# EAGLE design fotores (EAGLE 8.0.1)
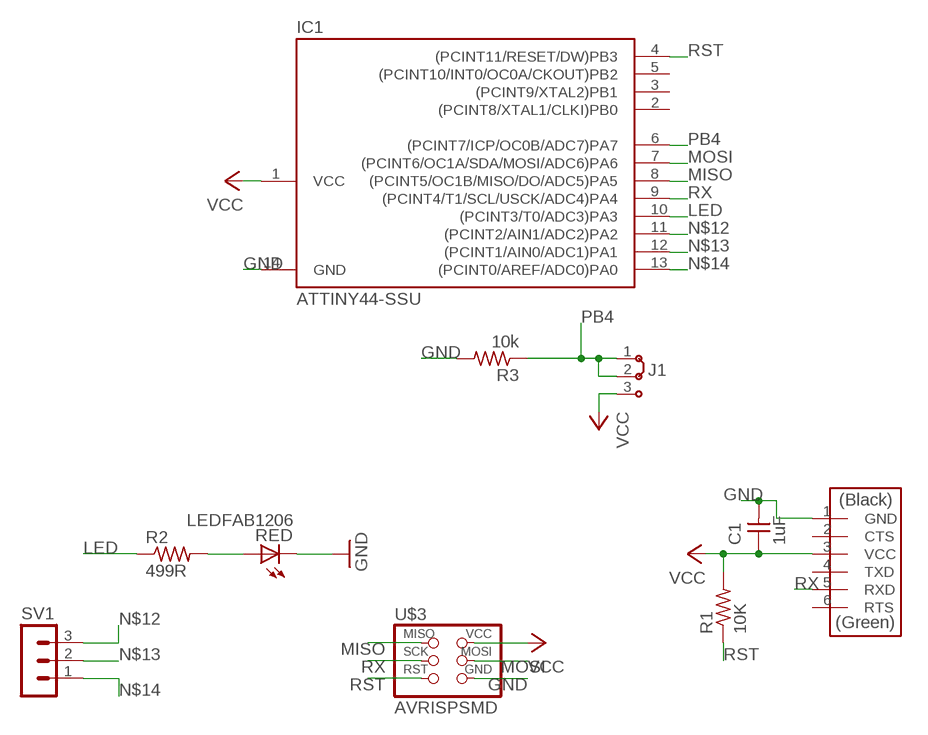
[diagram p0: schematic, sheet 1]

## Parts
C1  1uF  CAP-UNPOLARIZEDFAB  [C1206FAB]
IC1  ATTINY44-SSU  [SOIC14]
J1  J2X2MM  [04C]
R1  10K  RES-US1206FAB  [R1206FAB]
R2  499R  RES-US1206FAB  [R1206FAB]
R3  10k  RES-US1206FAB  [R1206FAB]
RED  LEDFAB1206  [LED1206FAB]
SV1  MA03-1  [MA03-1]
U$2  FTDI-SMD-HEADER  [1X06SMD]
U$3  AVRISPSMD  [2X03SMD]

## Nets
GND: C1.2 IC1.14(GND) R3.2 RED.2(C) U$2.1(GND) U$3.6(GND)
LED: IC1.10((PCINT3/T0/ADC3)PA3) R2.1
MISO: IC1.8((PCINT5/OC1B/MISO/DO/ADC5)PA5) U$3.1(MISO)
MOSI: IC1.7((PCINT6/OC1A/SDA/MOSI/ADC6)PA6) U$3.4(MOSI)
N$1: R2.2 RED.1(A)
N$12: IC1.11((PCINT2/AIN1/ADC2)PA2) SV1.3
N$13: IC1.12((PCINT1/AIN0/ADC1)PA1) SV1.2
N$14: IC1.13((PCINT0/AREF/ADC0)PA0) SV1.1
PB4: IC1.6((PCINT7/ICP/OC0B/ADC7)PA7) J1.1 J1.2 R3.1
RST: IC1.4((PCINT11/RESET/DW)PB3) R1.1 U$3.5(RST)
RX: IC1.9((PCINT4/T1/SCL/USCK/ADC4)PA4) U$2.5(RXD) U$3.3(SCK)
VCC: C1.1 IC1.1(VCC) J1.3 R1.2 U$2.3(VCC) U$3.2(VCC)
Unconnected: IC1.2((PCINT8/XTAL1/CLKI)PB0) IC1.3((PCINT9/XTAL2)PB1) IC1.5((PCINT10/INT0/OC0A/CKOUT)PB2) U$2.2(CTS) U$2.4(TXD) U$2.6(RTS)

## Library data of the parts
C1 = fab:CAP-UNPOLARIZED
IC1 = fab:ATTINY44
J1 = jumper:J2: Jumper switch 2 x 2.5 mm
R1-R3 = fab:RES-US: Resistor (US Symbol)
RED = fab:LED: LED
SV1 = con-lstb:MA03-1: PIN HEADER; OC_FARNELL: unknown; OC_NEWARK: unknown
U$2 = fab:FTDI-SMD-HEADER
U$3 = fab:AVRISP

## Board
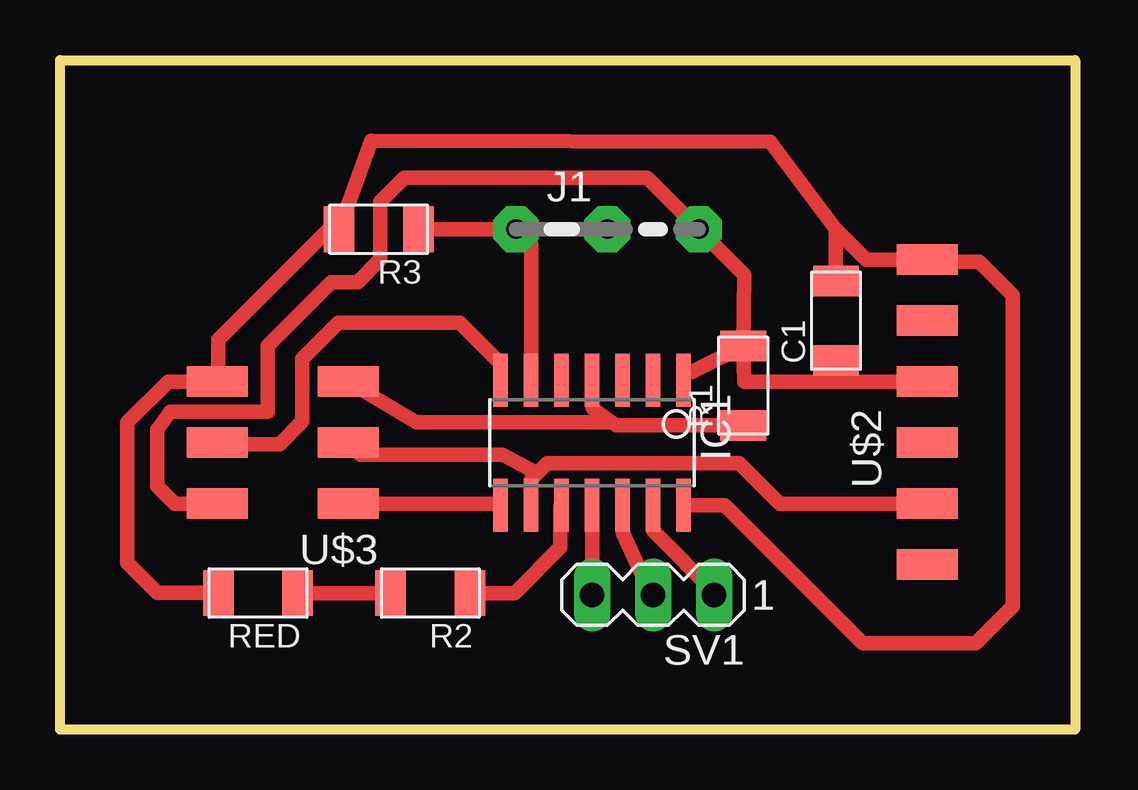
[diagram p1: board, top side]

Size 42.4 x 27.9 mm. Coordinates in mm from the lower left corner, seen from the top.
Outline: 0,0 42.4,0 42.4,27.8 0,27.8
Outline: 0,0 0,27.8
Outline: 0,27.8 0,27.9 42.3,27.9 42.3,0 0,0
Copper layers (1*16): Top 0.035mm / dielectric 1.5mm / Bottom 0.035mm
Design rules "default": minimum track width 10mil, minimum drill 24mil, track to track 8mil, track to pad 8mil, pad to pad 8mil, via to via 8mil, smd to smd 8mil, copper to edge 40mil, drill to drill 8mil, minimum pad ring 10mil, minimum via ring 8mil, stop-mask expansion 4mil, vias tented up to drill 0mil, thermal gap 10mil

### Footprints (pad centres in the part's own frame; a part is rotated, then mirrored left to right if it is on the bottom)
C1206FAB = smd 1.27 x 1.905: 1 -1.651,0; 2 1.651,0
SOIC14 = smd 0.61 x 2.21: 1 -3.81,-2.603; 2 -2.54,-2.603; 3 -1.27,-2.603; 4 0,-2.603; 5 1.27,-2.603; 6 2.54,-2.603; 7 3.81,-2.603; 8 3.81,2.603; 9 2.54,2.603; 10 1.27,2.603; 11 0,2.603; 12 -1.27,2.603; 13 -2.54,2.603; 14 -3.81,2.603
04C = drill 0.813 pad 1.905 octagon: 1 -1.905,0; 2 1.905,0; 3 5.715,0
R1206FAB = smd 1.27 x 1.905: 1 -1.651,0; 2 1.651,0
LED1206FAB = smd 1.27 x 1.905: 1 -1.651,0; 2 1.651,0
MA03-1 = drill 1.016 long: 1 -2.54,0; 2 0,0; 3 2.54,0
1X06SMD = smd 2.54 x 1.27: 1 0,6.35; 2 0,3.81; 3 0,1.27; 4 0,-1.27; 5 0,-3.81; 6 0,-6.35
2X03SMD = smd 2.54 x 1.27: 1 -2.54,2.54; 2 2.92,2.54; 3 -2.54,0; 4 2.92,0; 5 -2.54,-2.54; 6 2.92,-2.54

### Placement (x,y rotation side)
C1  32.33,17.04 90 top
IC1  22.17,11.96 180 top
J1  20.9,20.85 0 top
R1  28.47,14.33 90 top
R2  15.43,5.69 180 top
R3  13.28,20.85 180 top
RED  8.25,5.69 180 top
SV1  24.71,5.61 180 top
U$2  36.14,13.23 0 top
U$3  9.47,11.96 180 top

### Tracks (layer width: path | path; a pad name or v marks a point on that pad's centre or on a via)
GND
  Top 0.406: R3.2 11.2,20.85 | 6.6,14.55 U$3.6 | 6.59,5.7 RED.2
  Top 0.61: R3.2 12.97,24.54 29.59,24.49 32.33,20.85 | 32.33,20.85 33.6,19.58 U$2.1 36.22,19.5 38.3,19.5 39.7,18.1 39.7,5.15 38.15,3.6 33.45,3.6 27.69,9.36 IC1.14 | C1.2 32.33,20.85 | 11.2,20.85 6.6,16.25 6.6,14.55 | U$3.6 4.5,14.5 2.8,12.8 2.8,6.95 4.05,5.7 6.59,5.7
LED
  Top 0.406: 20.85,9.31 IC1.10
  Top 0.61: R2.1 18.94,5.69 20.85,7.6 20.85,9.31
MISO
  Top 0.406: 18.3,9.42 IC1.8
  Top 0.61: U$3.1 18.3,9.42
MOSI
  Top 0.406: IC1.7 18.36,15.24 | 6.61,11.9 U$3.4
  Top 0.61: 18.36,15.24 16.65,16.95 11.6,16.95 10.1,15.45 10.1,12.85 9.15,11.9 6.61,11.9
N$1
  Top 0.61: RED.1 R2.2
N$12
  Top 0.61: IC1.11 SV1.3
N$13
  Top 0.406: IC1.12 23.44,8.21 | 24.65,5.67 SV1.2
  Top 0.61: 23.44,8.21 24.6,5.7 24.65,5.67
N$14
  Top 0.406: 27.2,5.66 SV1.1
  Top 0.61: 27.2,5.66 27.35,5.65 24.71,8.29 IC1.13
PB4
  Top 0.406: 19.63,20.21 J1.1 J1.2
  Top 0.61: IC1.6 19.63,20.21 | R3.1 J1.1
RST
  Top 0.406: 22.99,12.82 23.17,12.68 | 22.2,13.4 22.2,14.53 IC1.4
  Top 0.61: R1.1 23.17,12.68 | 22.2,13.4 22.99,12.82 14.84,12.82 U$3.5
RX
  Top 0.406: 19.65,10.45 19.65,9.38 IC1.9 | 12.51,11.46 U$3.3
  Top 0.61: U$2.5 29.98,9.42 28.3,11.1 20.3,11.1 19.88,10.67 | 19.88,10.67 19.65,10.45 | 19.88,10.67 18.44,11.46 12.51,11.46
VCC
  Top 0.406: 26.3,14.88 IC1.1
  Top 0.61: 32.33,14.5 U$2.3 | 32.33,14.5 28.52,14.5 R1.2 | C1.1 32.33,14.5 | R1.2 28.52,18.95 J1.3 24.46,23 14.35,23 13.35,22 13.35,19.6 12.4,18.65 11.3,18.65 8.65,16 8.65,13.25 4.6,13.25 4.05,12.5 4.05,10.15 4.78,9.42 U$3.2 | R1.2 26.3,14.88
